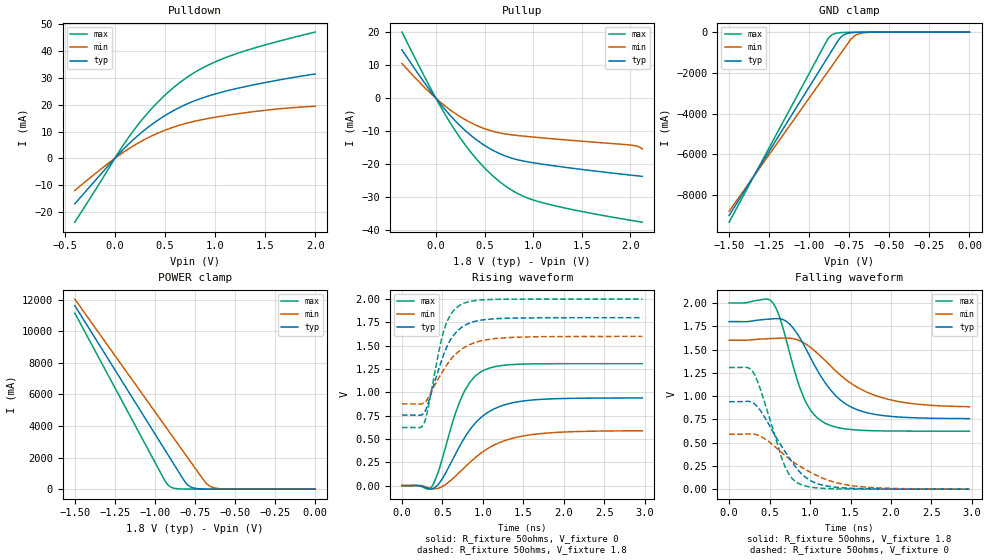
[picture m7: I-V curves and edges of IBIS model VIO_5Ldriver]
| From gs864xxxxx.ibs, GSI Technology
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|  signals   DQA1-DQA9, DQB1-DQB9, DQC1-DQC9, DQD1-DQD9
[Model]   VIO_5Ldriver
Model_type   I/O
Polarity   Non-Inverting
Vinl  =   0.75v
Vinh  =   1.75v
Vmeas =   0.9v
Cref  =   0pF
Rref  =   50
Vref  =   0.9v
|  variable   typ   min   max
C_comp   3.0pF   2.5pF   3.5pF
|  variable   typ   min   max
[Temperature Range]   50   0   100
|  variable   typ   min   max
[Voltage Range]   1.8   1.6   2.0
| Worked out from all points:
|   slope of the pulldown table from 0 to 0.27 V, typ, clamps not added: 27.7 ohm
|   slope of the pullup table from 0 to 0.27 V, typ, clamps not added: 30.3 ohm
|   GND clamp passes 1 mA (typ) near -0.58 V on its own axis
|   POWER clamp passes 1 mA (typ) near -0.61 V on its own axis
|   rising waveform, R_fixture 50ohms, V_fixture 0: 20-80 % time 435ps typ, 553ps min, 305ps max; typ from 0 V to 0.94 V
|   rising waveform, R_fixture 50ohms, V_fixture 1.8: 20-80 % time 269ps typ, 355ps min, 203ps max; typ from 0.756 V to 1.8 V
|   falling waveform, R_fixture 50ohms, V_fixture 1.8: 20-80 % time 468ps typ, 646ps min, 304ps max; typ from 1.8 V to 0.758 V
|   falling waveform, R_fixture 50ohms, V_fixture 0: 20-80 % time 416ps typ, 611ps min, 285ps max; typ from 0.94 V to 0 V
[Pulldown]
| voltage   typ   min   max
-400mV    -16.98mA   -11.98mA   -23.83mA
-50mV     -2.094mA   -1.415mA   -3.058mA
75mV      3.006mA    2.013mA    4.421mA
175mV     6.653mA    4.442mA    9.783mA
275mV     9.912mA    6.595mA    14.59mA
400mV     13.48mA    8.917mA    19.87mA
525mV     16.52mA    10.85mA    24.44mA
625mV     18.61mA    12.13mA    27.6mA
850mV     22.23mA    14.27mA    33.24mA
1.125V    25.27mA    16.09mA    37.89mA
1.5V      28.29mA    17.95mA    42.34mA
2V        31.52mA    19.45mA    47.14mA
[Pullup]
| voltage (VDDQ-Vout) typ   min   max
-350mV    14.7mA     10.57mA    20.08mA
-25mV     969.4uA    670.1uA    1.367mA
175mV     -6.111mA   -4.131mA   -8.754mA
400mV     -12.2mA    -8.004mA   -17.84mA
525mV     -14.75mA   -9.477mA   -21.86mA
650mV     -16.72mA   -10.48mA   -25.17mA
850mV     -18.73mA   -11.33mA   -29.04mA
1.05V     -19.79mA   -11.9mA    -31.31mA
1.475V    -21.5mA    -12.97mA   -34.2mA
2V        -23.3mA    -14.19mA   -37mA
2.075V    -23.54mA   -14.58mA   -37.36mA
2.125V    -23.7mA    -15.38mA   -37.6mA
[GND Clamp]
| voltage   typ   min   max
-1.5V     -9.007A    -8.796A    -9.334A
-900mV    -1.426A    -2.122A    -562.9mA
-880mV    -1.174A    -1.9A      -292.9mA
-860mV    -921.1mA   -1.678A    -142.5mA
-820mV    -416.2mA   -1.233A    -38.58mA
-800mV    -222mA     -1.011A    -23.51mA
-780mV    -116.3mA   -788.8mA   -16.2mA
-740mV    -33.04mA   -348.7mA   -9.876mA
-720mV    -18.57mA   -198.2mA   -8.142mA
-680mV    -6.87mA    -61.92mA   -5.539mA
-580mV    -1.002mA   -3.885mA   -1.438mA
0V        -402.5pA   -791.6pA   -356.8pA
[POWER Clamp]
| voltage (VDDQ-Vout) typ   min   max
-1.5V     11.62A     12.03A     11.14A
-940mV    2.526A     4.049A     574.2mA
-920mV    2.201A     3.764A     270.7mA
-900mV    1.877A     3.479A     123.3mA
-880mV    1.552A     3.194A     56.51mA
-820mV    578.6mA    2.34A      8.04mA
-800mV    303.9mA    2.055A     5.265mA
-760mV    77.74mA    1.486A     2.987mA
-680mV    5.757mA    367.3mA    1.268mA
-640mV    1.972mA    111.8mA    748.9uA
-540mV    239.3uA    5.502mA    108.9uA
0V        575.4pA    0A         0A
[Ramp]
| voltage   typ   min   max
dV/dt_r   1.53/137p   1.35/170p   1.77/112p
dV/dt_f   1.51/136p   1.31/167p   1.77/112p
R_load  =   50ohms
[Rising Waveform]
C_fixture =   0.0pf
R_fixture =   50ohms
V_fixture =   0
| Time   V(typ)   V(min)   V(max)
0s        6.524nV    16.51nV    4.386nV
360ps     -38.46mV   -29.4mV    -22.19mV
480ps     49.29mV    -18.88mV   233.7mV
630ps     285.4mV    76.51mV    692.2mV
750ps     479.8mV    175.2mV    972.7mV
900ps     663.8mV    295mV      1.17V
1.02ns    760.5mV    375.1mV    1.24V
1.26ns    863.7mV    478.9mV    1.29V
1.62ns    918.3mV    548.1mV    1.305V
2.97ns    939.5mV    588mV      1.307V
[Rising Waveform]
C_fixture =   0.0pf
R_fixture =   50ohms
V_fixture =   1.8
V_fixture_min =   1.6
V_fixture_max =   2.0
| Time   V(typ)   V(min)   V(max)
0s        755.9mV    876.3mV    622.9mV
270ps     775.6mV    885.5mV    659.2mV
300ps     821.9mV    905.9mV    735.5mV
480ps     1.317V     1.191V     1.537V
540ps     1.459V     1.275V     1.722V
630ps     1.602V     1.38V      1.868V
750ps     1.705V     1.47V      1.95V
960ps     1.771V     1.548V     1.989V
1.29ns    1.794V     1.586V     1.998V
2.97ns    1.8V       1.6V       2V
[Falling Waveform]
C_fixture =   0.0pf
R_fixture =   50ohms
V_fixture =   1.8
V_fixture_min =   1.6
V_fixture_max =   2.0
| Time   V(typ)   V(min)   V(max)
0s        1.8V       1.6V       2V
540ps     1.83V      1.619V     2.003V
630ps     1.83V      1.622V     1.831V
720ps     1.794V     1.623V     1.556V
930ps     1.538V     1.568V     966.9mV
1.17ns    1.165V     1.395V     716.4mV
1.38ns    953.8mV    1.221V     655.1mV
1.68ns    826.3mV    1.051V     630.6mV
2.19ns    770.6mV    927.2mV    623.9mV
2.97ns    757.9mV    884.9mV    623.2mV
[Falling Waveform]
C_fixture =   0.0pf
R_fixture =   50ohms
V_fixture =   0
| Time   V(typ)   V(min)   V(max)
0s        939.8mV    589.4mV    1.307V
210ps     943.9mV    591.8mV    1.309V
300ps     926.5mV    593.1mV    1.253V
390ps     840.5mV    568.1mV    1.064V
690ps     405.7mV    363.3mV    243.5mV
780ps     287.6mV    300.6mV    112.7mV
870ps     187.2mV    248.7mV    56.75mV
1.11ns    53.45mV    136mV      11.52mV
1.5ns     9.816mV    39.73mV    1.096mV
2.97ns    37.29uV    712.7uV    237.7nV
